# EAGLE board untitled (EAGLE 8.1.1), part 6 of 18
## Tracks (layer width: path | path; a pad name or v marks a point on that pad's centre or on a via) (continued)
S$5547 (continued)
  Bottom 0: 104.1,93.68 104.19,93.45
S$5548
  Bottom 0: 104.19,93.45 56.98,93.45
S$5549
  Bottom 0: 93.36,96.09 95.24,96.09
S$5550
  Bottom 0: 95.24,96.09 95.32,96.1
S$5551
  Bottom 0: 95.32,96.1 95.39,96.14
S$5552
  Bottom 0: 95.39,96.14 95.44,96.19
S$5553
  Bottom 0: 95.44,96.19 95.48,96.27
S$5554
  Bottom 0: 95.48,96.27 95.49,96.34
S$5555
  Bottom 0: 95.49,96.34 95.49,98.22
S$5556
  Bottom 0: 95.49,98.22 95.48,98.3
S$5557
  Bottom 0: 95.48,98.3 95.44,98.37
S$5558
  Bottom 0: 95.44,98.37 95.39,98.42
S$5559
  Bottom 0: 95.39,98.42 95.32,98.47
S$5560
  Bottom 0: 95.32,98.47 95.24,98.48
S$5561
  Bottom 0: 95.24,98.48 93.36,98.48
S$5562
  Bottom 0: 93.36,98.48 93.28,98.47
S$5563
  Bottom 0: 93.28,98.47 93.21,98.42
S$5564
  Bottom 0: 93.21,98.42 93.16,98.37
S$5565
  Bottom 0: 93.16,98.37 93.12,98.3
S$5566
  Bottom 0: 93.12,98.3 93.1,98.22
S$5567
  Bottom 0: 93.1,98.22 93.1,96.34
S$5568
  Bottom 0: 93.1,96.34 93.12,96.27
S$5569
  Bottom 0: 93.12,96.27 93.16,96.19
S$5570
  Bottom 0: 93.16,96.19 93.21,96.14
S$5571
  Bottom 0: 93.21,96.14 93.28,96.1
S$5572
  Bottom 0: 93.28,96.1 93.36,96.09
S$5573
  Bottom 0: 98.59,96.1 98.91,96.12
S$5574
  Bottom 0: 98.91,96.12 99.22,96.22
S$5575
  Bottom 0: 99.22,96.22 99.48,96.41
S$5576
  Bottom 0: 99.48,96.41 99.69,96.67
S$5577
  Bottom 0: 99.69,96.67 99.82,96.97
S$5578
  Bottom 0: 99.82,96.97 99.86,97.29
S$5579
  Bottom 0: 99.86,97.29 99.82,97.61
S$5580
  Bottom 0: 99.82,97.61 99.69,97.91
S$5581
  Bottom 0: 99.69,97.91 99.48,98.16
S$5582
  Bottom 0: 99.48,98.16 99.22,98.35
S$5583
  Bottom 0: 99.22,98.35 98.91,98.45
S$5584
  Bottom 0: 98.91,98.45 98.59,98.48
S$5585
  Bottom 0: 98.59,98.48 98.27,98.41
S$5586
  Bottom 0: 98.27,98.41 97.98,98.26
S$5587
  Bottom 0: 97.98,98.26 97.74,98.04
S$5588
  Bottom 0: 97.74,98.04 97.57,97.77
S$5589
  Bottom 0: 97.57,97.77 97.48,97.45
S$5590
  Bottom 0: 97.48,97.45 97.48,97.12
S$5591
  Bottom 0: 97.48,97.12 97.57,96.81
S$5592
  Bottom 0: 97.57,96.81 97.74,96.53
S$5593
  Bottom 0: 97.74,96.53 97.98,96.31
S$5594
  Bottom 0: 97.98,96.31 98.27,96.16
S$5595
  Bottom 0: 98.27,96.16 98.59,96.1
S$5596
  Bottom 0: 104.8,109.99 105.15,110.05
S$5597
  Bottom 0: 105.15,110.05 105.46,110.2
S$5598
  Bottom 0: 105.46,110.2 105.73,110.42
S$5599
  Bottom 0: 105.73,110.42 105.94,110.71
S$5600
  Bottom 0: 105.94,110.71 106.06,111.03
S$5601
  Bottom 0: 106.06,111.03 106.11,111.38
S$5602
  Bottom 0: 106.11,111.38 106.06,111.72
S$5603
  Bottom 0: 106.06,111.72 105.94,112.05
S$5604
  Bottom 0: 105.94,112.05 105.73,112.33
S$5605
  Bottom 0: 105.73,112.33 105.46,112.56
S$5606
  Bottom 0: 105.46,112.56 105.15,112.71
S$5607
  Bottom 0: 105.15,112.71 104.8,112.77
S$5608
  Bottom 0: 104.8,112.77 104.45,112.75
S$5609
  Bottom 0: 104.45,112.75 104.12,112.64
S$5610
  Bottom 0: 104.12,112.64 104.09,112.63
S$5611
  Bottom 0: 104.09,112.63 103.53,113.2
S$5612
  Bottom 0: 103.53,113.2 103.47,113.24
S$5613
  Bottom 0: 103.47,113.24 103.41,113.28
S$5614
  Bottom 0: 103.41,113.28 103.35,113.3
S$5615
  Bottom 0: 103.35,113.3 103.28,113.32
S$5616
  Bottom 0: 103.28,113.32 103.21,113.33
S$5617
  Bottom 0: 103.21,113.33 98.64,113.33
S$5618
  Bottom 0: 98.64,113.33 98.57,113.46
S$5619
  Bottom 0: 98.57,113.46 98.37,113.67
S$5620
  Bottom 0: 98.37,113.67 98.11,113.83
S$5621
  Bottom 0: 98.11,113.83 97.81,113.89
S$5622
  Bottom 0: 97.81,113.89 97.51,113.87
S$5623
  Bottom 0: 97.51,113.87 97.23,113.76
S$5624
  Bottom 0: 97.23,113.76 96.99,113.57
S$5625
  Bottom 0: 96.99,113.57 96.82,113.33
S$5626
  Bottom 0: 96.82,113.33 96.73,113.03
S$5627
  Bottom 0: 96.73,113.03 96.73,112.73
S$5628
  Bottom 0: 96.73,112.73 96.82,112.44
S$5629
  Bottom 0: 96.82,112.44 96.99,112.19
S$5630
  Bottom 0: 96.99,112.19 97.23,112
S$5631
  Bottom 0: 97.23,112 97.51,111.89
S$5632
  Bottom 0: 97.51,111.89 97.81,111.87
S$5633
  Bottom 0: 97.81,111.87 98.11,111.94
S$5634
  Bottom 0: 98.11,111.94 98.37,112.09
S$5635
  Bottom 0: 98.37,112.09 98.57,112.31
S$5636
  Bottom 0: 98.57,112.31 98.64,112.44
S$5637
  Bottom 0: 98.64,112.44 103.02,112.44
S$5638
  Bottom 0: 103.02,112.44 103.47,111.99
S$5639
  Bottom 0: 103.47,111.99 103.41,111.89
S$5640
  Bottom 0: 103.41,111.89 103.33,111.55
S$5641
  Bottom 0: 103.33,111.55 103.33,111.21
S$5642
  Bottom 0: 103.33,111.21 103.41,110.87
S$5643
  Bottom 0: 103.41,110.87 103.59,110.56
S$5644
  Bottom 0: 103.59,110.56 103.83,110.3
S$5645
  Bottom 0: 103.83,110.3 104.12,110.11
S$5646
  Bottom 0: 104.12,110.11 104.45,110.01
S$5647
  Bottom 0: 104.45,110.01 104.8,109.99
S$5648
  Bottom 0: 85.75,109.99 86.09,110.05
S$5649
  Bottom 0: 86.09,110.05 86.4,110.2
S$5650
  Bottom 0: 86.4,110.2 86.67,110.42
S$5651
  Bottom 0: 86.67,110.42 86.88,110.71
S$5652
  Bottom 0: 86.88,110.71 87.01,111.03
S$5653
  Bottom 0: 87.01,111.03 87.06,111.38
S$5654
  Bottom 0: 87.06,111.38 87.01,111.72
S$5655
  Bottom 0: 87.01,111.72 86.88,112.05
S$5656
  Bottom 0: 86.88,112.05 86.67,112.33
S$5657
  Bottom 0: 86.67,112.33 86.4,112.56
S$5658
  Bottom 0: 86.4,112.56 86.09,112.71
S$5659
  Bottom 0: 86.09,112.71 85.75,112.77
S$5660
  Bottom 0: 85.75,112.77 85.39,112.75
S$5661
  Bottom 0: 85.39,112.75 85.06,112.64
S$5662
  Bottom 0: 85.06,112.64 85.04,112.63
S$5663
  Bottom 0: 85.04,112.63 84.47,113.2
S$5664
  Bottom 0: 84.47,113.2 84.41,113.24
S$5665
  Bottom 0: 84.41,113.24 84.35,113.28
S$5666
  Bottom 0: 84.35,113.28 84.29,113.3
S$5667
  Bottom 0: 84.29,113.3 84.23,113.32
S$5668
  Bottom 0: 84.23,113.32 84.16,113.33
S$5669
  Bottom 0: 84.16,113.33 79.58,113.33
S$5670
  Bottom 0: 79.58,113.33 79.52,113.46
S$5671
  Bottom 0: 79.52,113.46 79.31,113.67
S$5672
  Bottom 0: 79.31,113.67 79.05,113.83
S$5673
  Bottom 0: 79.05,113.83 78.75,113.89
S$5674
  Bottom 0: 78.75,113.89 78.45,113.87
S$5675
  Bottom 0: 78.45,113.87 78.17,113.76
S$5676
  Bottom 0: 78.17,113.76 77.93,113.57
S$5677
  Bottom 0: 77.93,113.57 77.76,113.33
S$5678
  Bottom 0: 77.76,113.33 77.67,113.03
S$5679
  Bottom 0: 77.67,113.03 77.67,112.73
S$5680
  Bottom 0: 77.67,112.73 77.76,112.44
S$5681
  Bottom 0: 77.76,112.44 77.93,112.19
S$5682
  Bottom 0: 77.93,112.19 78.17,112
S$5683
  Bottom 0: 78.17,112 78.45,111.89
S$5684
  Bottom 0: 78.45,111.89 78.75,111.87
S$5685
  Bottom 0: 78.75,111.87 79.05,111.94
S$5686
  Bottom 0: 79.05,111.94 79.31,112.09
S$5687
  Bottom 0: 79.31,112.09 79.52,112.31
S$5688
  Bottom 0: 79.52,112.31 79.58,112.44
S$5689
  Bottom 0: 79.58,112.44 83.97,112.44
S$5690
  Bottom 0: 83.97,112.44 84.41,111.99
S$5691
  Bottom 0: 84.41,111.99 84.36,111.89
S$5692
  Bottom 0: 84.36,111.89 84.27,111.55
S$5693
  Bottom 0: 84.27,111.55 84.27,111.21
S$5694
  Bottom 0: 84.27,111.21 84.36,110.87
S$5695
  Bottom 0: 84.36,110.87 84.53,110.56
S$5696
  Bottom 0: 84.53,110.56 84.77,110.3
S$5697
  Bottom 0: 84.77,110.3 85.06,110.11
S$5698
  Bottom 0: 85.06,110.11 85.39,110.01
S$5699
  Bottom 0: 85.39,110.01 85.75,109.99
S$5700
  Bottom 0: 73.05,112.53 73.39,112.59
S$5701
  Bottom 0: 73.39,112.59 73.7,112.74
S$5702
  Bottom 0: 73.7,112.74 73.97,112.96
S$5703
  Bottom 0: 73.97,112.96 74.18,113.25
S$5704
  Bottom 0: 74.18,113.25 74.31,113.57
S$5705
  Bottom 0: 74.31,113.57 74.36,113.92
S$5706
  Bottom 0: 74.36,113.92 74.31,114.26
S$5707
  Bottom 0: 74.31,114.26 74.18,114.59
S$5708
  Bottom 0: 74.18,114.59 73.97,114.87
S$5709
  Bottom 0: 73.97,114.87 73.7,115.1
S$5710
  Bottom 0: 73.7,115.1 73.39,115.25
S$5711
  Bottom 0: 73.39,115.25 73.05,115.31
S$5712
  Bottom 0: 73.05,115.31 72.69,115.29
S$5713
  Bottom 0: 72.69,115.29 72.36,115.18
S$5714
  Bottom 0: 72.36,115.18 72.07,115
S$5715
  Bottom 0: 72.07,115 71.83,114.74
S$5716
  Bottom 0: 71.83,114.74 71.66,114.43
S$5717
  Bottom 0: 71.66,114.43 71.57,114.09
S$5718
  Bottom 0: 71.57,114.09 71.57,113.75
S$5719
  Bottom 0: 71.57,113.75 71.66,113.41
S$5720
  Bottom 0: 71.66,113.41 71.83,113.1
S$5721
  Bottom 0: 71.83,113.1 72.07,112.84
S$5722
  Bottom 0: 72.07,112.84 72.36,112.65
S$5723
  Bottom 0: 72.36,112.65 72.69,112.55
S$5724
  Bottom 0: 72.69,112.55 73.05,112.53
S$5725
  Bottom 0: 92.09,112.53 92.44,112.59
S$5726
  Bottom 0: 92.44,112.59 92.75,112.74
S$5727
  Bottom 0: 92.75,112.74 93.03,112.96
S$5728
  Bottom 0: 93.03,112.96 93.23,113.25
S$5729
  Bottom 0: 93.23,113.25 93.36,113.57
S$5730
  Bottom 0: 93.36,113.57 93.41,113.92
S$5731
  Bottom 0: 93.41,113.92 93.36,114.26
S$5732
  Bottom 0: 93.36,114.26 93.23,114.59
S$5733
  Bottom 0: 93.23,114.59 93.03,114.87
S$5734
  Bottom 0: 93.03,114.87 92.75,115.1
S$5735
  Bottom 0: 92.75,115.1 92.44,115.25
S$5736
  Bottom 0: 92.44,115.25 92.09,115.31
S$5737
  Bottom 0: 92.09,115.31 91.75,115.29
S$5738
  Bottom 0: 91.75,115.29 91.42,115.18
S$5739
  Bottom 0: 91.42,115.18 91.12,115
S$5740
  Bottom 0: 91.12,115 90.88,114.74
S$5741
  Bottom 0: 90.88,114.74 90.71,114.43
S$5742
  Bottom 0: 90.71,114.43 90.62,114.09
S$5743
  Bottom 0: 90.62,114.09 90.62,113.75
S$5744
  Bottom 0: 90.62,113.75 90.71,113.41
S$5745
  Bottom 0: 90.71,113.41 90.88,113.1
S$5746
  Bottom 0: 90.88,113.1 91.12,112.84
S$5747
  Bottom 0: 91.12,112.84 91.42,112.65
S$5748
  Bottom 0: 91.42,112.65 91.75,112.55
S$5749
  Bottom 0: 91.75,112.55 92.09,112.53
S$5750
  Bottom 0: 88.2,114.17 88.65,114.22
S$5751
  Bottom 0: 88.65,114.22 89.07,114.35
S$5752
  Bottom 0: 89.07,114.35 89.47,114.56
S$5753
  Bottom 0: 89.47,114.56 89.81,114.84
S$5754
  Bottom 0: 89.81,114.84 90.1,115.19
S$5755
  Bottom 0: 90.1,115.19 90.31,115.58
S$5756
  Bottom 0: 90.31,115.58 90.44,116.01
S$5757
  Bottom 0: 90.44,116.01 90.48,116.46
S$5758
  Bottom 0: 90.48,116.46 90.44,116.91
S$5759
  Bottom 0: 90.44,116.91 90.31,117.33
S$5760
  Bottom 0: 90.31,117.33 90.1,117.73
S$5761
  Bottom 0: 90.1,117.73 89.81,118.07
S$5762
  Bottom 0: 89.81,118.07 89.47,118.36
S$5763
  Bottom 0: 89.47,118.36 89.07,118.57
S$5764
  Bottom 0: 89.07,118.57 88.65,118.7
S$5765
  Bottom 0: 88.65,118.7 88.2,118.75
S$5766
  Bottom 0: 88.2,118.75 87.75,118.7
S$5767
  Bottom 0: 87.75,118.7 87.32,118.57
S$5768
  Bottom 0: 87.32,118.57 86.93,118.36
S$5769
  Bottom 0: 86.93,118.36 86.58,118.07
S$5770
  Bottom 0: 86.58,118.07 86.3,117.73
S$5771
  Bottom 0: 86.3,117.73 86.08,117.33
S$5772
  Bottom 0: 86.08,117.33 85.96,116.91
S$5773
  Bottom 0: 85.96,116.91 85.91,116.46
S$5774
  Bottom 0: 85.91,116.46 85.96,116.01
S$5775
  Bottom 0: 85.96,116.01 86.08,115.58
S$5776
  Bottom 0: 86.08,115.58 86.3,115.19
S$5777
  Bottom 0: 86.3,115.19 86.58,114.84
S$5778
  Bottom 0: 86.58,114.84 86.93,114.56
S$5779
  Bottom 0: 86.93,114.56 87.32,114.35
S$5780
  Bottom 0: 87.32,114.35 87.75,114.22
S$5781
  Bottom 0: 87.75,114.22 88.2,114.17
S$5782
  Bottom 0: 88.28,138.54 88.58,138.61
S$5783
  Bottom 0: 88.58,138.61 88.84,138.76
S$5784
  Bottom 0: 88.84,138.76 89.05,138.98
S$5785
  Bottom 0: 89.05,138.98 89.18,139.25
S$5786
  Bottom 0: 89.18,139.25 89.22,139.55
S$5787
  Bottom 0: 89.22,139.55 89.18,139.85
S$5788
  Bottom 0: 89.18,139.85 89.05,140.13
S$5789
  Bottom 0: 89.05,140.13 88.84,140.34
S$5790
  Bottom 0: 88.84,140.34 88.58,140.5
S$5791
  Bottom 0: 88.58,140.5 88.28,140.56
S$5792
  Bottom 0: 88.28,140.56 87.98,140.54
S$5793
  Bottom 0: 87.98,140.54 87.7,140.43
S$5794
  Bottom 0: 87.7,140.43 87.46,140.24
S$5795
  Bottom 0: 87.46,140.24 87.29,140
S$5796
  Bottom 0: 87.29,140 87.2,139.71
S$5797
  Bottom 0: 87.2,139.71 87.2,139.4
S$5798
  Bottom 0: 87.2,139.4 87.29,139.11
S$5799
  Bottom 0: 87.29,139.11 87.46,138.86
S$5800
  Bottom 0: 87.46,138.86 87.7,138.67
S$5801
  Bottom 0: 87.7,138.67 87.98,138.56
S$5802
  Bottom 0: 87.98,138.56 88.28,138.54
S$5803
  Bottom 0: 90.51,148.09 90.86,148.15
S$5804
  Bottom 0: 90.86,148.15 91.17,148.3
S$5805
  Bottom 0: 91.17,148.3 91.44,148.52
S$5806
  Bottom 0: 91.44,148.52 91.65,148.81
S$5807
  Bottom 0: 91.65,148.81 91.78,149.13
S$5808
  Bottom 0: 91.78,149.13 91.82,149.48
S$5809
  Bottom 0: 91.82,149.48 91.78,149.82
S$5810
  Bottom 0: 91.78,149.82 91.65,150.15
S$5811
  Bottom 0: 91.65,150.15 91.44,150.43
S$5812
  Bottom 0: 91.44,150.43 91.17,150.66
S$5813
  Bottom 0: 91.17,150.66 90.86,150.81
S$5814
  Bottom 0: 90.86,150.81 90.51,150.87
S$5815
  Bottom 0: 90.51,150.87 90.16,150.85
S$5816
  Bottom 0: 90.16,150.85 89.83,150.74
S$5817
  Bottom 0: 89.83,150.74 89.53,150.56
S$5818
  Bottom 0: 89.53,150.56 89.29,150.3
S$5819
  Bottom 0: 89.29,150.3 89.12,149.99
S$5820
  Bottom 0: 89.12,149.99 89.04,149.65
S$5821
  Bottom 0: 89.04,149.65 89.04,149.3
S$5822
  Bottom 0: 89.04,149.3 89.12,148.97
S$5823
  Bottom 0: 89.12,148.97 89.29,148.66
S$5824
  Bottom 0: 89.29,148.66 89.53,148.4
S$5825
  Bottom 0: 89.53,148.4 89.83,148.21
S$5826
  Bottom 0: 89.83,148.21 90.16,148.11
S$5827
  Bottom 0: 90.16,148.11 90.51,148.09
S$5828
  Bottom 0: 246.64,93.68 239.2,101.12
S$5829
  Bottom 0: 239.2,101.12 239.21,101.15
S$5830
  Bottom 0: 239.21,101.15 239.26,101.45
S$5831
  Bottom 0: 239.26,101.45 239.21,101.75
S$5832
  Bottom 0: 239.21,101.75 239.08,102.02
S$5833
  Bottom 0: 239.08,102.02 238.88,102.24
S$5834
  Bottom 0: 238.88,102.24 238.61,102.39
S$5835
  Bottom 0: 238.61,102.39 238.32,102.46
S$5836
  Bottom 0: 238.32,102.46 238.08,102.44
S$5837
  Bottom 0: 238.08,102.44 246.78,111.14
S$5838
  Bottom 0: 246.78,111.14 246.82,111.19
S$5839
  Bottom 0: 246.82,111.19 246.86,111.25
S$5840
  Bottom 0: 246.86,111.25 246.88,111.31
S$5841
  Bottom 0: 246.88,111.31 246.9,111.38
S$5842
  Bottom 0: 246.9,111.38 246.9,111.45
S$5843
  Bottom 0: 246.9,111.45 246.9,138.72
S$5844
  Bottom 0: 246.9,138.72 246.97,138.78
S$5845
  Bottom 0: 246.97,138.78 247.1,138.99
S$5846
  Bottom 0: 247.1,138.99 247.15,139.24
S$5847
  Bottom 0: 247.15,139.24 247.1,139.49
S$5848
  Bottom 0: 247.1,139.49 246.97,139.7
S$5849
  Bottom 0: 246.97,139.7 246.77,139.85
S$5850
  Bottom 0: 246.77,139.85 246.52,139.92
S$5851
  Bottom 0: 246.52,139.92 246.27,139.9
S$5852
  Bottom 0: 246.27,139.9 246.05,139.78
S$5853
  Bottom 0: 246.05,139.78 245.88,139.6
S$5854
  Bottom 0: 245.88,139.6 245.79,139.37
S$5855
  Bottom 0: 245.79,139.37 245.79,139.11
S$5856
  Bottom 0: 245.79,139.11 245.88,138.88
S$5857
  Bottom 0: 245.88,138.88 246.02,138.72
S$5858
  Bottom 0: 246.02,138.72 246.02,111.64
S$5859
  Bottom 0: 246.02,111.64 229.12,94.74
S$5860
  Bottom 0: 229.12,94.74 229.14,94.87
S$5861
  Bottom 0: 229.14,94.87 229.09,95.21
S$5862
  Bottom 0: 229.09,95.21 228.97,95.54
S$5863
  Bottom 0: 228.97,95.54 228.75,95.82
S$5864
  Bottom 0: 228.75,95.82 228.49,96.05
S$5865
  Bottom 0: 228.49,96.05 228.18,96.19
S$5866
  Bottom 0: 228.18,96.19 228.18,97.27
S$5867
  Bottom 0: 228.18,97.27 228.18,97.34
S$5868
  Bottom 0: 228.18,97.34 228.16,97.41
S$5869
  Bottom 0: 228.16,97.41 228.14,97.47
S$5870
  Bottom 0: 228.14,97.47 228.1,97.53
S$5871
  Bottom 0: 228.1,97.53 228.05,97.59
S$5872
  Bottom 0: 228.05,97.59 225.4,100.25
S$5873
  Bottom 0: 225.4,100.25 243.96,118.81
S$5874
  Bottom 0: 243.96,118.81 244,118.87
S$5875
  Bottom 0: 244,118.87 244.04,118.93
S$5876
  Bottom 0: 244.04,118.93 244.06,118.99
S$5877
  Bottom 0: 244.06,118.99 244.08,119.06
S$5878
  Bottom 0: 244.08,119.06 244.08,119.13
S$5879
  Bottom 0: 244.08,119.13 244.08,140.04
S$5880
  Bottom 0: 244.08,140.04 244.08,140.12
S$5881
  Bottom 0: 244.08,140.12 244.06,140.18
S$5882
  Bottom 0: 244.06,140.18 244.04,140.24
S$5883
  Bottom 0: 244.04,140.24 244,140.31
S$5884
  Bottom 0: 244,140.31 243.96,140.36
S$5885
  Bottom 0: 243.96,140.36 231.98,152.33
S$5886
  Bottom 0: 231.98,152.33 231.93,152.38
S$5887
  Bottom 0: 231.93,152.38 231.86,152.41
S$5888
  Bottom 0: 231.86,152.41 231.8,152.44
S$5889
  Bottom 0: 231.8,152.44 231.74,152.46
S$5890
  Bottom 0: 231.74,152.46 231.67,152.46
S$5891
  Bottom 0: 231.67,152.46 231.44,152.46
S$5892
  Bottom 0: 231.44,152.46 231.35,152.69
S$5893
  Bottom 0: 231.35,152.69 231.14,152.97
S$5894
  Bottom 0: 231.14,152.97 230.87,153.2
S$5895
  Bottom 0: 230.87,153.2 230.56,153.35
S$5896
  Bottom 0: 230.56,153.35 230.21,153.41
S$5897
  Bottom 0: 230.21,153.41 229.86,153.39
S$5898
  Bottom 0: 229.86,153.39 229.53,153.28
S$5899
  Bottom 0: 229.53,153.28 229.24,153.1
S$5900
  Bottom 0: 229.24,153.1 229,152.84
S$5901
  Bottom 0: 229,152.84 228.82,152.53
S$5902
  Bottom 0: 228.82,152.53 228.8,152.46
S$5903
  Bottom 0: 228.8,152.46 227.22,152.46
S$5904
  Bottom 0: 227.22,152.46 227.58,152.66
S$5905
  Bottom 0: 227.58,152.66 227.93,152.94
S$5906
  Bottom 0: 227.93,152.94 228.21,153.29
S$5907
  Bottom 0: 228.21,153.29 228.43,153.68
S$5908
  Bottom 0: 228.43,153.68 228.55,154.11
S$5909
  Bottom 0: 228.55,154.11 228.6,154.56
S$5910
  Bottom 0: 228.6,154.56 228.55,155.01
S$5911
  Bottom 0: 228.55,155.01 228.43,155.43
S$5912
  Bottom 0: 228.43,155.43 228.21,155.83
S$5913
  Bottom 0: 228.21,155.83 227.93,156.17
S$5914
  Bottom 0: 227.93,156.17 227.58,156.46
S$5915
  Bottom 0: 227.58,156.46 227.19,156.67
S$5916
  Bottom 0: 227.19,156.67 226.76,156.8
S$5917
  Bottom 0: 226.76,156.8 226.31,156.84
S$5918
  Bottom 0: 226.31,156.84 225.87,156.8
S$5919
  Bottom 0: 225.87,156.8 225.44,156.67
S$5920
  Bottom 0: 225.44,156.67 225.04,156.46
S$5921
  Bottom 0: 225.04,156.46 224.7,156.17
S$5922
  Bottom 0: 224.7,156.17 224.41,155.83
S$5923
  Bottom 0: 224.41,155.83 224.2,155.43
S$5924
  Bottom 0: 224.2,155.43 224.07,155.01
S$5925
  Bottom 0: 224.07,155.01 224.03,154.56
S$5926
  Bottom 0: 224.03,154.56 224.07,154.11
S$5927
  Bottom 0: 224.07,154.11 224.2,153.68
S$5928
  Bottom 0: 224.2,153.68 224.41,153.29
S$5929
  Bottom 0: 224.41,153.29 224.7,152.94
S$5930
  Bottom 0: 224.7,152.94 225.04,152.66
S$5931
  Bottom 0: 225.04,152.66 225.41,152.46
S$5932
  Bottom 0: 225.41,152.46 217.72,152.46
S$5933
  Bottom 0: 217.72,152.46 211.52,158.66
S$5934
  Bottom 0: 211.52,158.66 211.47,158.7
S$5935
  Bottom 0: 211.47,158.7 211.4,158.74
S$5936
  Bottom 0: 211.4,158.74 211.34,158.76
S$5937
  Bottom 0: 211.34,158.76 211.28,158.78
S$5938
  Bottom 0: 211.28,158.78 211.21,158.79
S$5939
  Bottom 0: 211.21,158.79 209.29,158.79
S$5940
  Bottom 0: 209.29,158.79 209.49,159.02
S$5941
  Bottom 0: 209.49,159.02 209.63,159.32
S$5942
  Bottom 0: 209.63,159.32 209.68,159.64
S$5943
  Bottom 0: 209.68,159.64 209.63,159.96
S$5944
  Bottom 0: 209.63,159.96 209.49,160.26
S$5945
  Bottom 0: 209.49,160.26 209.28,160.5
S$5946
  Bottom 0: 209.28,160.5 209.1,160.62
S$5947
  Bottom 0: 209.1,160.62 209.1,161.66
S$5948
  Bottom 0: 209.1,161.66 209.1,161.75
S$5949
  Bottom 0: 209.1,161.75 209.08,161.84
S$5950
  Bottom 0: 209.08,161.84 209.04,161.92
S$5951
  Bottom 0: 209.04,161.92 209,162
S$5952
  Bottom 0: 209,162 208.94,162.06
S$5953
  Bottom 0: 208.94,162.06 201.29,169.7
S$5954
  Bottom 0: 201.29,169.7 201.63,169.68
S$5955
  Bottom 0: 201.63,169.68 201.98,169.74
S$5956
  Bottom 0: 201.98,169.74 202.16,169.83
S$5957
  Bottom 0: 202.16,169.83 205.24,166.75
S$5958
  Bottom 0: 205.24,166.75 205.29,166.71
S$5959
  Bottom 0: 205.29,166.71 205.35,166.66
S$5960
  Bottom 0: 205.35,166.66 205.41,166.64
S$5961
  Bottom 0: 205.41,166.64 205.48,166.62
S$5962
  Bottom 0: 205.48,166.62 205.55,166.62
S$5963
  Bottom 0: 205.55,166.62 208.77,166.62
S$5964
  Bottom 0: 208.77,166.62 211.33,164.06
S$5965
  Bottom 0: 211.33,164.06 211.01,164.08
S$5966
  Bottom 0: 211.01,164.08 210.69,164.02
S$5967
  Bottom 0: 210.69,164.02 210.4,163.87
S$5968
  Bottom 0: 210.4,163.87 210.17,163.65
S$5969
  Bottom 0: 210.17,163.65 210,163.37
S$5970
  Bottom 0: 210,163.37 209.91,163.06
S$5971
  Bottom 0: 209.91,163.06 209.91,162.73
S$5972
  Bottom 0: 209.91,162.73 210,162.42
S$5973
  Bottom 0: 210,162.42 210.17,162.14
S$5974
  Bottom 0: 210.17,162.14 210.4,161.92
S$5975
  Bottom 0: 210.4,161.92 210.69,161.77
S$5976
  Bottom 0: 210.69,161.77 211.01,161.71
S$5977
  Bottom 0: 211.01,161.71 211.34,161.73
S$5978
  Bottom 0: 211.34,161.73 211.64,161.83
S$5979
  Bottom 0: 211.64,161.83 211.91,162.02
S$5980
  Bottom 0: 211.91,162.02 212.11,162.28
S$5981
  Bottom 0: 212.11,162.28 212.24,162.57
S$5982
  Bottom 0: 212.24,162.57 212.29,162.89
S$5983
  Bottom 0: 212.29,162.89 212.24,163.22
S$5984
  Bottom 0: 212.24,163.22 212.23,163.25
S$5985
  Bottom 0: 212.23,163.25 212.28,163.24
S$5986
  Bottom 0: 212.28,163.24 212.35,163.23
S$5987
  Bottom 0: 212.35,163.23 213.16,163.23
S$5988
  Bottom 0: 213.16,163.23 216.78,159.61
S$5989
  Bottom 0: 216.78,159.61 216.58,159.59
S$5990
  Bottom 0: 216.58,159.59 216.3,159.48
S$5991
  Bottom 0: 216.3,159.48 216.06,159.29
S$5992
  Bottom 0: 216.06,159.29 215.89,159.04
S$5993
  Bottom 0: 215.89,159.04 215.8,158.75
S$5994
  Bottom 0: 215.8,158.75 215.8,158.45
S$5995
  Bottom 0: 215.8,158.45 215.89,158.16
S$5996
  Bottom 0: 215.89,158.16 216.06,157.91
S$5997
  Bottom 0: 216.06,157.91 216.3,157.72
S$5998
  Bottom 0: 216.3,157.72 216.58,157.61
S$5999
  Bottom 0: 216.58,157.61 216.88,157.59
S$6000
  Bottom 0: 216.88,157.59 217.18,157.66
S$6001
  Bottom 0: 217.18,157.66 217.44,157.81
S$6002
  Bottom 0: 217.44,157.81 217.64,158.03
S$6003
  Bottom 0: 217.64,158.03 217.78,158.3
S$6004
  Bottom 0: 217.78,158.3 217.81,158.57
S$6005
  Bottom 0: 217.81,158.57 218.98,157.4
S$6006
  Bottom 0: 218.98,157.4 219.03,157.36
S$6007
  Bottom 0: 219.03,157.36 219.09,157.32
S$6008
  Bottom 0: 219.09,157.32 219.16,157.29
S$6009
  Bottom 0: 219.16,157.29 219.22,157.28
S$6010
  Bottom 0: 219.22,157.28 219.29,157.27
S$6011
  Bottom 0: 219.29,157.27 235.43,157.27
S$6012
  Bottom 0: 235.43,157.27 241,151.7
S$6013
  Bottom 0: 241,151.7 241.05,151.66
S$6014
  Bottom 0: 241.05,151.66 241.11,151.62
S$6015
  Bottom 0: 241.11,151.62 241.17,151.6
S$6016
  Bottom 0: 241.17,151.6 241.24,151.58
S$6017
  Bottom 0: 241.24,151.58 241.31,151.58
S$6018
  Bottom 0: 241.31,151.58 247.85,151.58
S$6019
  Bottom 0: 247.85,151.58 247.87,151.51
S$6020
  Bottom 0: 247.87,151.51 248.05,151.2
S$6021
  Bottom 0: 248.05,151.2 248.28,150.94
S$6022
  Bottom 0: 248.28,150.94 248.58,150.75
S$6023
  Bottom 0: 248.58,150.75 248.91,150.65
S$6024
  Bottom 0: 248.91,150.65 249.26,150.63
S$6025
  Bottom 0: 249.26,150.63 249.61,150.69
S$6026
  Bottom 0: 249.61,150.69 249.79,150.77
S$6027
  Bottom 0: 249.79,150.77 249.88,150.68
S$6028
  Bottom 0: 249.88,150.68 249.94,150.63
S$6029
  Bottom 0: 249.94,150.63 250,150.6
S$6030
  Bottom 0: 250,150.6 250.06,150.57
S$6031
  Bottom 0: 250.06,150.57 250.13,150.56
S$6032
  Bottom 0: 250.13,150.56 250.2,150.55
S$6033
  Bottom 0: 250.2,150.55 252.78,150.55
S$6034
  Bottom 0: 252.78,150.55 253.72,149.61
S$6035
  Bottom 0: 253.72,149.61 253.5,149.6
S$6036
  Bottom 0: 253.5,149.6 253.22,149.48
S$6037
  Bottom 0: 253.22,149.48 252.98,149.3
S$6038
  Bottom 0: 252.98,149.3 252.81,149.04
S$6039
  Bottom 0: 252.81,149.04 244.14,149.04
S$6040
  Bottom 0: 244.14,149.04 244.18,149.13
S$6041
  Bottom 0: 244.18,149.13 244.22,149.48
S$6042
  Bottom 0: 244.22,149.48 244.18,149.82
S$6043
  Bottom 0: 244.18,149.82 244.05,150.15
S$6044
  Bottom 0: 244.05,150.15 243.84,150.43
S$6045
  Bottom 0: 243.84,150.43 243.57,150.66
S$6046
  Bottom 0: 243.57,150.66 243.26,150.81
S$6047
  Bottom 0: 243.26,150.81 242.91,150.87
S$6048
  Bottom 0: 242.91,150.87 242.56,150.85
S$6049
  Bottom 0: 242.56,150.85 242.23,150.74
S$6050
  Bottom 0: 242.23,150.74 241.94,150.56
S$6051
  Bottom 0: 241.94,150.56 241.7,150.3
S$6052
  Bottom 0: 241.7,150.3 241.52,149.99
S$6053
  Bottom 0: 241.52,149.99 241.44,149.65
S$6054
  Bottom 0: 241.44,149.65 241.44,149.3
S$6055
  Bottom 0: 241.44,149.3 241.52,148.97
S$6056
  Bottom 0: 241.52,148.97 241.7,148.66
S$6057
  Bottom 0: 241.7,148.66 241.94,148.4
S$6058
  Bottom 0: 241.94,148.4 242.23,148.21
S$6059
  Bottom 0: 242.23,148.21 242.56,148.11
S$6060
  Bottom 0: 242.56,148.11 242.91,148.09
S$6061
  Bottom 0: 242.91,148.09 243.26,148.15
S$6062
  Bottom 0: 243.26,148.15 243.45,148.25
S$6063
  Bottom 0: 243.45,148.25 243.5,148.21
S$6064
  Bottom 0: 243.5,148.21 243.56,148.18
S$6065
  Bottom 0: 243.56,148.18 243.63,148.17
S$6066
  Bottom 0: 243.63,148.17 243.7,148.16
S$6067
  Bottom 0: 243.7,148.16 252.81,148.16
S$6068
  Bottom 0: 252.81,148.16 252.98,147.91
S$6069
  Bottom 0: 252.98,147.91 253.22,147.73
S$6070
  Bottom 0: 253.22,147.73 253.5,147.62
S$6071
  Bottom 0: 253.5,147.62 253.8,147.59
S$6072
  Bottom 0: 253.8,147.59 254.1,147.66
S$6073
  Bottom 0: 254.1,147.66 254.36,147.81
S$6074
  Bottom 0: 254.36,147.81 254.56,148.03
S$6075
  Bottom 0: 254.56,148.03 254.7,148.31
S$6076
  Bottom 0: 254.7,148.31 254.74,148.59
S$6077
  Bottom 0: 254.74,148.59 257.62,145.71
S$6078
  Bottom 0: 257.62,145.71 248.02,136.09
S$6079
  Bottom 0: 248.02,136.09 247.97,136.03
S$6080
  Bottom 0: 247.97,136.03 247.93,135.97
S$6081
  Bottom 0: 247.93,135.97 247.91,135.91
S$6082
  Bottom 0: 247.91,135.91 247.89,135.85
S$6083
  Bottom 0: 247.89,135.85 247.89,135.78
S$6084
  Bottom 0: 247.89,135.78 247.89,127
S$6085
  Bottom 0: 247.89,127 247.75,126.84
S$6086
  Bottom 0: 247.75,126.84 247.66,126.61
S$6087
  Bottom 0: 247.66,126.61 247.66,126.36
S$6088
  Bottom 0: 247.66,126.36 247.75,126.12
S$6089
  Bottom 0: 247.75,126.12 247.89,125.97
S$6090
  Bottom 0: 247.89,125.97 247.89,109.06
S$6091
  Bottom 0: 247.89,109.06 244.91,106.09
S$6092
  Bottom 0: 244.91,106.09 244.86,106.03
S$6093
  Bottom 0: 244.86,106.03 244.83,105.97
S$6094
  Bottom 0: 244.83,105.97 244.79,105.91
S$6095
  Bottom 0: 244.79,105.91 244.78,105.84
S$6096
  Bottom 0: 244.78,105.84 244.78,105.77
S$6097
  Bottom 0: 244.78,105.77 244.78,101.33
S$6098
  Bottom 0: 244.78,101.33 244.78,101.25
S$6099
  Bottom 0: 244.78,101.25 244.79,101.19
S$6100
  Bottom 0: 244.79,101.19 244.83,101.12
S$6101
  Bottom 0: 244.83,101.12 244.86,101.07
S$6102
  Bottom 0: 244.86,101.07 244.91,101.01
S$6103
  Bottom 0: 244.91,101.01 245.57,100.34
S$6104
  Bottom 0: 245.57,100.34 245.63,100.3
S$6105
  Bottom 0: 245.63,100.3 245.69,100.26
S$6106
  Bottom 0: 245.69,100.26 245.75,100.24
S$6107
  Bottom 0: 245.75,100.24 245.82,100.22
S$6108
  Bottom 0: 245.82,100.22 245.89,100.22
S$6109
  Bottom 0: 245.89,100.22 247.83,100.22
S$6110
  Bottom 0: 247.83,100.22 248.48,99.56
S$6111
  Bottom 0: 248.48,99.56 248.19,99.65
S$6112
  Bottom 0: 248.19,99.65 247.75,99.69
S$6113
  Bottom 0: 247.75,99.69 247.3,99.65
S$6114
  Bottom 0: 247.3,99.65 246.87,99.52
S$6115
  Bottom 0: 246.87,99.52 246.48,99.31
S$6116
  Bottom 0: 246.48,99.31 246.13,99.02
S$6117
  Bottom 0: 246.13,99.02 245.85,98.68
S$6118
  Bottom 0: 245.85,98.68 245.63,98.28
S$6119
  Bottom 0: 245.63,98.28 245.51,97.86
S$6120
  Bottom 0: 245.51,97.86 245.46,97.41
S$6121
  Bottom 0: 245.46,97.41 245.51,96.96
S$6122
  Bottom 0: 245.51,96.96 245.63,96.53
S$6123
  Bottom 0: 245.63,96.53 245.85,96.14
S$6124
  Bottom 0: 245.85,96.14 246.13,95.79
S$6125
  Bottom 0: 246.13,95.79 246.48,95.51
S$6126
  Bottom 0: 246.48,95.51 246.87,95.3
S$6127
  Bottom 0: 246.87,95.3 247.3,95.17
S$6128
  Bottom 0: 247.3,95.17 247.75,95.12
S$6129
  Bottom 0: 247.75,95.12 248.19,95.17
S$6130
  Bottom 0: 248.19,95.17 248.62,95.3
S$6131
  Bottom 0: 248.62,95.3 249.02,95.51
S$6132
  Bottom 0: 249.02,95.51 249.36,95.79
S$6133
  Bottom 0: 249.36,95.79 249.64,96.14
S$6134
  Bottom 0: 249.64,96.14 249.86,96.53
S$6135
  Bottom 0: 249.86,96.53 249.99,96.96
S$6136
  Bottom 0: 249.99,96.96 250.03,97.41
S$6137
  Bottom 0: 250.03,97.41 249.99,97.86
S$6138
  Bottom 0: 249.99,97.86 249.9,98.15
S$6139
  Bottom 0: 249.9,98.15 251.12,96.93
S$6140
  Bottom 0: 251.12,96.93 251.12,96.19
S$6141
  Bottom 0: 251.12,96.19 250.96,96.13
S$6142
  Bottom 0: 250.96,96.13 250.67,95.95
S$6143
  Bottom 0: 250.67,95.95 250.43,95.69
S$6144
  Bottom 0: 250.43,95.69 250.26,95.38
S$6145
  Bottom 0: 250.26,95.38 250.17,95.04
S$6146
  Bottom 0: 250.17,95.04 250.17,94.7
S$6147
  Bottom 0: 250.17,94.7 250.26,94.36
S$6148
  Bottom 0: 250.26,94.36 250.43,94.05
S$6149
  Bottom 0: 250.43,94.05 250.67,93.79
S$6150
  Bottom 0: 250.67,93.79 250.84,93.68
S$6151
  Bottom 0: 250.84,93.68 246.64,93.68
S$6152
  Bottom 0: 252.28,93.68 252.3,93.69
S$6153
  Bottom 0: 252.3,93.69 252.57,93.91
S$6154
  Bottom 0: 252.57,93.91 252.78,94.2
S$6155
  Bottom 0: 252.78,94.2 252.91,94.52
S$6156
  Bottom 0: 252.91,94.52 252.95,94.87
S$6157
  Bottom 0: 252.95,94.87 252.91,95.21
S$6158
  Bottom 0: 252.91,95.21 252.78,95.54
S$6159
  Bottom 0: 252.78,95.54 252.57,95.82
S$6160
  Bottom 0: 252.57,95.82 252.3,96.05
S$6161
  Bottom 0: 252.3,96.05 252,96.19
S$6162
  Bottom 0: 252,96.19 252,97.12
S$6163
  Bottom 0: 252,97.12 251.99,97.19
S$6164
  Bottom 0: 251.99,97.19 251.98,97.26
S$6165
  Bottom 0: 251.98,97.26 251.95,97.32
S$6166
  Bottom 0: 251.95,97.32 251.91,97.38
S$6167
  Bottom 0: 251.91,97.38 251.87,97.43
S$6168
  Bottom 0: 251.87,97.43 248.53,100.78
S$6169
  Bottom 0: 248.53,100.78 254.93,100.78
S$6170
  Bottom 0: 254.93,100.78 255,100.78
S$6171
  Bottom 0: 255,100.78 255.06,100.8
S$6172
  Bottom 0: 255.06,100.8 255.12,100.82
S$6173
  Bottom 0: 255.12,100.82 255.18,100.86
S$6174
  Bottom 0: 255.18,100.86 255.24,100.9
S$6175
  Bottom 0: 255.24,100.9 255.65,101.31
S$6176
  Bottom 0: 255.65,101.31 255.71,101.28
S$6177
  Bottom 0: 255.71,101.28 256.03,101.21
S$6178
  Bottom 0: 256.03,101.21 256.35,101.23
S$6179
  Bottom 0: 256.35,101.23 256.66,101.34
S$6180
  Bottom 0: 256.66,101.34 256.92,101.53
S$6181
  Bottom 0: 256.92,101.53 257.13,101.78
S$6182
  Bottom 0: 257.13,101.78 257.26,102.08
S$6183
  Bottom 0: 257.26,102.08 257.3,102.4
S$6184
  Bottom 0: 257.3,102.4 257.26,102.72
S$6185
  Bottom 0: 257.26,102.72 257.13,103.02
S$6186
  Bottom 0: 257.13,103.02 256.92,103.28
S$6187
  Bottom 0: 256.92,103.28 256.66,103.46
S$6188
  Bottom 0: 256.66,103.46 256.35,103.57
S$6189
  Bottom 0: 256.35,103.57 256.03,103.59
S$6190
  Bottom 0: 256.03,103.59 255.71,103.53
S$6191
  Bottom 0: 255.71,103.53 255.42,103.38
S$6192
  Bottom 0: 255.42,103.38 255.18,103.15
S$6193
  Bottom 0: 255.18,103.15 255.01,102.88
S$6194
  Bottom 0: 255.01,102.88 254.93,102.56
S$6195
  Bottom 0: 254.93,102.56 254.93,102.24
S$6196
  Bottom 0: 254.93,102.24 255.01,101.94
S$6197
  Bottom 0: 255.01,101.94 254.74,101.66
S$6198
  Bottom 0: 254.74,101.66 249.79,101.66
S$6199
  Bottom 0: 249.79,101.66 249.98,101.87
S$6200
  Bottom 0: 249.98,101.87 250.11,102.17
S$6201
  Bottom 0: 250.11,102.17 250.16,102.49
S$6202
  Bottom 0: 250.16,102.49 250.11,102.81
S$6203
  Bottom 0: 250.11,102.81 249.98,103.11
S$6204
  Bottom 0: 249.98,103.11 249.76,103.35
S$6205
  Bottom 0: 249.76,103.35 249.58,103.47
S$6206
  Bottom 0: 249.58,103.47 249.58,111.78
S$6207
  Bottom 0: 249.58,111.78 255.18,117.38
S$6208
  Bottom 0: 255.18,117.38 255.16,117.33
S$6209
  Bottom 0: 255.16,117.33 255.03,116.91
S$6210
  Bottom 0: 255.03,116.91 254.99,116.46
S$6211
  Bottom 0: 254.99,116.46 255.03,116.01
S$6212
  Bottom 0: 255.03,116.01 255.16,115.58
S$6213
  Bottom 0: 255.16,115.58 255.37,115.19
S$6214
  Bottom 0: 255.37,115.19 255.66,114.84
S$6215
  Bottom 0: 255.66,114.84 256,114.56
S$6216
  Bottom 0: 256,114.56 256.4,114.35
S$6217
  Bottom 0: 256.4,114.35 256.82,114.22
S$6218
  Bottom 0: 256.82,114.22 257.27,114.17
S$6219
  Bottom 0: 257.27,114.17 257.72,114.22
S$6220
  Bottom 0: 257.72,114.22 258.14,114.35
S$6221
  Bottom 0: 258.14,114.35 258.54,114.56
S$6222
  Bottom 0: 258.54,114.56 258.89,114.84
S$6223
  Bottom 0: 258.89,114.84 259.17,115.19
S$6224
  Bottom 0: 259.17,115.19 259.38,115.58
S$6225
  Bottom 0: 259.38,115.58 259.51,116.01
S$6226
  Bottom 0: 259.51,116.01 259.56,116.46
S$6227
  Bottom 0: 259.56,116.46 259.51,116.91
S$6228
  Bottom 0: 259.51,116.91 259.38,117.33
S$6229
  Bottom 0: 259.38,117.33 259.17,117.73
S$6230
  Bottom 0: 259.17,117.73 258.89,118.07
S$6231
  Bottom 0: 258.89,118.07 258.54,118.36
S$6232
  Bottom 0: 258.54,118.36 258.14,118.57
S$6233
  Bottom 0: 258.14,118.57 257.72,118.7
S$6234
  Bottom 0: 257.72,118.7 257.27,118.75
S$6235
  Bottom 0: 257.27,118.75 256.82,118.7
S$6236
  Bottom 0: 256.82,118.7 256.4,118.57
S$6237
  Bottom 0: 256.4,118.57 256.35,118.55
S$6238
  Bottom 0: 256.35,118.55 258.25,120.45
S$6239
  Bottom 0: 258.25,120.45 258.38,120.41
S$6240
  Bottom 0: 258.38,120.41 258.7,120.41
S$6241
  Bottom 0: 258.7,120.41 259.01,120.5
S$6242
  Bottom 0: 259.01,120.5 259.29,120.67
S$6243
  Bottom 0: 259.29,120.67 259.5,120.92
S$6244
  Bottom 0: 259.5,120.92 259.64,121.22
S$6245
  Bottom 0: 259.64,121.22 259.69,121.54
S$6246
  Bottom 0: 259.69,121.54 259.64,121.86
S$6247
  Bottom 0: 259.64,121.86 259.5,122.16
S$6248
  Bottom 0: 259.5,122.16 259.29,122.4
S$6249
  Bottom 0: 259.29,122.4 259.01,122.58
S$6250
  Bottom 0: 259.01,122.58 258.7,122.67
S$6251
  Bottom 0: 258.7,122.67 258.38,122.67
S$6252
  Bottom 0: 258.38,122.67 258.25,122.63
S$6253
  Bottom 0: 258.25,122.63 258.2,122.68
S$6254
  Bottom 0: 258.2,122.68 258.2,129.9
S$6255
  Bottom 0: 258.2,129.9 258.36,129.61
S$6256
  Bottom 0: 258.36,129.61 258.6,129.35
S$6257
  Bottom 0: 258.6,129.35 258.9,129.16
S$6258
  Bottom 0: 258.9,129.16 259.23,129.06
S$6259
  Bottom 0: 259.23,129.06 259.58,129.04
S$6260
  Bottom 0: 259.58,129.04 259.92,129.1
S$6261
  Bottom 0: 259.92,129.1 260.24,129.25
S$6262
  Bottom 0: 260.24,129.25 260.5,129.47
S$6263
  Bottom 0: 260.5,129.47 260.72,129.76
S$6264
  Bottom 0: 260.72,129.76 260.84,130.08
S$6265
  Bottom 0: 260.84,130.08 260.89,130.43
S$6266
  Bottom 0: 260.89,130.43 260.84,130.77
S$6267
  Bottom 0: 260.84,130.77 260.72,131.1
S$6268
  Bottom 0: 260.72,131.1 260.5,131.38
S$6269
  Bottom 0: 260.5,131.38 260.24,131.61
S$6270
  Bottom 0: 260.24,131.61 259.92,131.76
S$6271
  Bottom 0: 259.92,131.76 259.58,131.82
S$6272
  Bottom 0: 259.58,131.82 259.23,131.8
S$6273
  Bottom 0: 259.23,131.8 258.9,131.69
S$6274
  Bottom 0: 258.9,131.69 258.6,131.51
S$6275
  Bottom 0: 258.6,131.51 258.36,131.25
S$6276
  Bottom 0: 258.36,131.25 258.2,130.96
S$6277
  Bottom 0: 258.2,130.96 258.2,134.69
S$6278
  Bottom 0: 258.2,134.69 259.94,136.43
S$6279
  Bottom 0: 259.94,136.43 259.92,136.38
S$6280
  Bottom 0: 259.92,136.38 259.79,135.96
S$6281
  Bottom 0: 259.79,135.96 259.74,135.51
S$6282
  Bottom 0: 259.74,135.51 259.79,135.06
S$6283
  Bottom 0: 259.79,135.06 259.92,134.63
S$6284
  Bottom 0: 259.92,134.63 260.13,134.24
S$6285
  Bottom 0: 260.13,134.24 260.42,133.89
S$6286
  Bottom 0: 260.42,133.89 260.76,133.61
S$6287
  Bottom 0: 260.76,133.61 261.16,133.4
S$6288
  Bottom 0: 261.16,133.4 261.58,133.27
S$6289
  Bottom 0: 261.58,133.27 262.03,133.22
S$6290
  Bottom 0: 262.03,133.22 262.48,133.27
S$6291
  Bottom 0: 262.48,133.27 262.9,133.4
S$6292
  Bottom 0: 262.9,133.4 263.3,133.61
S$6293
  Bottom 0: 263.3,133.61 263.65,133.89
S$6294
  Bottom 0: 263.65,133.89 263.93,134.24
S$6295
  Bottom 0: 263.93,134.24 264.14,134.63
S$6296
  Bottom 0: 264.14,134.63 264.27,135.06
S$6297
  Bottom 0: 264.27,135.06 264.31,135.51
S$6298
  Bottom 0: 264.31,135.51 264.27,135.96
S$6299
  Bottom 0: 264.27,135.96 264.14,136.38
S$6300
  Bottom 0: 264.14,136.38 263.93,136.78
S$6301
  Bottom 0: 263.93,136.78 263.65,137.12
S$6302
  Bottom 0: 263.65,137.12 263.3,137.41
S$6303
  Bottom 0: 263.3,137.41 262.9,137.62
S$6304
  Bottom 0: 262.9,137.62 262.48,137.75
S$6305
  Bottom 0: 262.48,137.75 262.03,137.79
S$6306
  Bottom 0: 262.03,137.79 261.58,137.75
S$6307
  Bottom 0: 261.58,137.75 261.16,137.62
S$6308
  Bottom 0: 261.16,137.62 261.11,137.6
S$6309
  Bottom 0: 261.11,137.6 263.01,139.5
S$6310
  Bottom 0: 263.01,139.5 263.14,139.46
S$6311
  Bottom 0: 263.14,139.46 263.46,139.46
S$6312
  Bottom 0: 263.46,139.46 263.77,139.55
S$6313
  Bottom 0: 263.77,139.55 264.05,139.72
S$6314
  Bottom 0: 264.05,139.72 264.26,139.97
S$6315
  Bottom 0: 264.26,139.97 264.4,140.27
S$6316
  Bottom 0: 264.4,140.27 264.44,140.59
S$6317
  Bottom 0: 264.44,140.59 264.4,140.91
S$6318
  Bottom 0: 264.4,140.91 264.26,141.21
S$6319
  Bottom 0: 264.26,141.21 264.05,141.45
S$6320
  Bottom 0: 264.05,141.45 263.77,141.63
S$6321
  Bottom 0: 263.77,141.63 263.46,141.72
S$6322
  Bottom 0: 263.46,141.72 263.14,141.72
S$6323
  Bottom 0: 263.14,141.72 262.83,141.63
S$6324
  Bottom 0: 262.83,141.63 262.56,141.45
S$6325
  Bottom 0: 262.56,141.45 262.34,141.21
S$6326
  Bottom 0: 262.34,141.21 262.2,140.91
S$6327
  Bottom 0: 262.2,140.91 262.16,140.59
S$6328
  Bottom 0: 262.16,140.59 262.2,140.29
S$6329
  Bottom 0: 262.2,140.29 261.9,140
S$6330
  Bottom 0: 261.9,140 261.9,141.48
S$6331
  Bottom 0: 261.9,141.48 261.89,141.55
S$6332
  Bottom 0: 261.89,141.55 261.85,141.62
S$6333
  Bottom 0: 261.85,141.62 261.8,141.68
S$6334
  Bottom 0: 261.8,141.68 261.73,141.72
S$6335
  Bottom 0: 261.73,141.72 261.65,141.73
S$6336
  Bottom 0: 261.65,141.73 261.2,141.73
S$6337
  Bottom 0: 261.2,141.73 261.2,141.86
S$6338
  Bottom 0: 261.2,141.86 261.14,142.08
S$6339
  Bottom 0: 261.14,142.08 260.98,142.24
S$6340
  Bottom 0: 260.98,142.24 260.76,142.3
S$6341
  Bottom 0: 260.76,142.3 260.43,142.3
S$6342
  Bottom 0: 260.43,142.3 259.34,143.39
S$6343
  Bottom 0: 259.34,143.39 259.4,143.52
S$6344
  Bottom 0: 259.4,143.52 259.45,143.84
S$6345
  Bottom 0: 259.45,143.84 259.44,143.88
S$6346
  Bottom 0: 259.44,143.88 261.24,142.08
S$6347
  Bottom 0: 261.24,142.08 261.3,142.04
S$6348
  Bottom 0: 261.3,142.04 261.36,142
S$6349
  Bottom 0: 261.36,142 261.42,141.97
S$6350
  Bottom 0: 261.42,141.97 261.48,141.96
S$6351
  Bottom 0: 261.48,141.96 261.55,141.95
S$6352
  Bottom 0: 261.55,141.95 279.15,141.95
S$6353
  Bottom 0: 279.15,141.95 279.21,141.96
S$6354
  Bottom 0: 279.21,141.96 261.04,123.78
S$6355
  Bottom 0: 261.04,123.78 261,123.72
S$6356
  Bottom 0: 261,123.72 260.95,123.66
S$6357
  Bottom 0: 260.95,123.66 260.93,123.6
S$6358
  Bottom 0: 260.93,123.6 260.91,123.53
S$6359
  Bottom 0: 260.91,123.53 260.91,123.46
S$6360
  Bottom 0: 260.91,123.46 260.91,118.07
S$6361
  Bottom 0: 260.91,118.07 260.86,118.11
S$6362
  Bottom 0: 260.86,118.11 260.61,118.18
S$6363
  Bottom 0: 260.61,118.18 260.37,118.16
S$6364
  Bottom 0: 260.37,118.16 260.14,118.04
S$6365
  Bottom 0: 260.14,118.04 259.97,117.86
S$6366
  Bottom 0: 259.97,117.86 259.88,117.62
S$6367
  Bottom 0: 259.88,117.62 259.88,117.37
S$6368
  Bottom 0: 259.88,117.37 259.97,117.14
S$6369
  Bottom 0: 259.97,117.14 260.11,116.99
S$6370
  Bottom 0: 260.11,116.99 260.11,115.95
S$6371
  Bottom 0: 260.11,115.95 259.18,115.02
S$6372
  Bottom 0: 259.18,115.02 259.14,114.97
S$6373
  Bottom 0: 259.14,114.97 259.1,114.91
S$6374
  Bottom 0: 259.1,114.91 259.07,114.84
S$6375
  Bottom 0: 259.07,114.84 259.06,114.78
S$6376
  Bottom 0: 259.06,114.78 259.05,114.71
S$6377
  Bottom 0: 259.05,114.71 259.05,113.26
S$6378
  Bottom 0: 259.05,113.26 259.06,113.2
S$6379
  Bottom 0: 259.06,113.2 259.07,113.13
S$6380
  Bottom 0: 259.07,113.13 259.1,113.07
S$6381
  Bottom 0: 259.1,113.07 259.13,113.01
S$6382
  Bottom 0: 259.13,113.01 259.18,112.95
S$6383
  Bottom 0: 259.18,112.95 259.26,112.87
S$6384
  Bottom 0: 259.26,112.87 259.26,103.99
S$6385
  Bottom 0: 259.26,103.99 259.12,104.14
S$6386
  Bottom 0: 259.12,104.14 258.93,104.26
S$6387
  Bottom 0: 258.93,104.26 258.93,107.62
S$6388
  Bottom 0: 258.93,107.62 258.92,107.7
S$6389
  Bottom 0: 258.92,107.7 258.91,107.76
S$6390
  Bottom 0: 258.91,107.76 258.88,107.82
S$6391
  Bottom 0: 258.88,107.82 258.84,107.88
S$6392
  Bottom 0: 258.84,107.88 258.8,107.94
S$6393
  Bottom 0: 258.8,107.94 255.98,110.76
S$6394
  Bottom 0: 255.98,110.76 256.08,111.03
S$6395
  Bottom 0: 256.08,111.03 256.13,111.38
S$6396
  Bottom 0: 256.13,111.38 256.08,111.72
S$6397
  Bottom 0: 256.08,111.72 255.96,112.05
S$6398
  Bottom 0: 255.96,112.05 255.75,112.33
S$6399
  Bottom 0: 255.75,112.33 255.48,112.56
S$6400
  Bottom 0: 255.48,112.56 255.16,112.71
S$6401
  Bottom 0: 255.16,112.71 254.82,112.77
S$6402
  Bottom 0: 254.82,112.77 254.47,112.75
S$6403
  Bottom 0: 254.47,112.75 254.14,112.64
S$6404
  Bottom 0: 254.14,112.64 253.84,112.46
S$6405
  Bottom 0: 253.84,112.46 253.6,112.2
S$6406
  Bottom 0: 253.6,112.2 253.43,111.89
S$6407
  Bottom 0: 253.43,111.89 253.34,111.55
S$6408
  Bottom 0: 253.34,111.55 253.34,111.21
S$6409
  Bottom 0: 253.34,111.21 253.43,110.87
S$6410
  Bottom 0: 253.43,110.87 253.6,110.56
S$6411
  Bottom 0: 253.6,110.56 253.84,110.3
S$6412
  Bottom 0: 253.84,110.3 254.14,110.11
S$6413
  Bottom 0: 254.14,110.11 254.47,110.01
S$6414
  Bottom 0: 254.47,110.01 254.82,109.99
S$6415
  Bottom 0: 254.82,109.99 255.16,110.05
S$6416
  Bottom 0: 255.16,110.05 255.35,110.13
S$6417
  Bottom 0: 255.35,110.13 258.04,107.44
S$6418
  Bottom 0: 258.04,107.44 258.04,104.26
S$6419
  Bottom 0: 258.04,104.26 257.98,104.23
S$6420
  Bottom 0: 257.98,104.23 257.74,104.04
S$6421
  Bottom 0: 257.74,104.04 257.57,103.8
S$6422
  Bottom 0: 257.57,103.8 257.48,103.5
S$6423
  Bottom 0: 257.48,103.5 257.48,103.2
S$6424
  Bottom 0: 257.48,103.2 257.57,102.91
S$6425
  Bottom 0: 257.57,102.91 257.74,102.66
S$6426
  Bottom 0: 257.74,102.66 257.98,102.47
S$6427
  Bottom 0: 257.98,102.47 258.26,102.36
S$6428
  Bottom 0: 258.26,102.36 258.56,102.34
S$6429
  Bottom 0: 258.56,102.34 258.85,102.41
S$6430
  Bottom 0: 258.85,102.41 259.12,102.56
S$6431
  Bottom 0: 259.12,102.56 259.26,102.71
S$6432
  Bottom 0: 259.26,102.71 259.26,97.14
S$6433
  Bottom 0: 259.26,97.14 258.81,96.69
S$6434
  Bottom 0: 258.81,96.69 258.56,96.74
S$6435
  Bottom 0: 258.56,96.74 258.26,96.72
S$6436
  Bottom 0: 258.26,96.72 257.98,96.61
S$6437
  Bottom 0: 257.98,96.61 257.74,96.42
S$6438
  Bottom 0: 257.74,96.42 257.57,96.17
S$6439
  Bottom 0: 257.57,96.17 257.48,95.89
S$6440
  Bottom 0: 257.48,95.89 257.48,95.58
S$6441
  Bottom 0: 257.48,95.58 257.57,95.29
S$6442
  Bottom 0: 257.57,95.29 257.74,95.04
S$6443
  Bottom 0: 257.74,95.04 257.98,94.85
S$6444
  Bottom 0: 257.98,94.85 258.26,94.74
S$6445
  Bottom 0: 258.26,94.74 258.56,94.72
S$6446
  Bottom 0: 258.56,94.72 258.85,94.79
S$6447
  Bottom 0: 258.85,94.79 259.12,94.94
S$6448
  Bottom 0: 259.12,94.94 259.32,95.16
S$6449
  Bottom 0: 259.32,95.16 259.46,95.43
S$6450
  Bottom 0: 259.46,95.43 259.5,95.73
S$6451
  Bottom 0: 259.5,95.73 259.46,96.03
S$6452
  Bottom 0: 259.46,96.03 259.44,96.06
S$6453
  Bottom 0: 259.44,96.06 260.02,96.65
S$6454
  Bottom 0: 260.02,96.65 260.06,96.7
S$6455
  Bottom 0: 260.06,96.7 260.1,96.76
S$6456
  Bottom 0: 260.1,96.76 260.12,96.82
S$6457
  Bottom 0: 260.12,96.82 260.14,96.89
S$6458
  Bottom 0: 260.14,96.89 260.15,96.96
S$6459
  Bottom 0: 260.15,96.96 260.15,112.89
S$6460
  Bottom 0: 260.15,112.89 260.19,112.84
S$6461
  Bottom 0: 260.19,112.84 260.49,112.65
S$6462
  Bottom 0: 260.49,112.65 260.81,112.55
S$6463
  Bottom 0: 260.81,112.55 261.17,112.53
S$6464
  Bottom 0: 261.17,112.53 261.51,112.59
S$6465
  Bottom 0: 261.51,112.59 261.7,112.67
S$6466
  Bottom 0: 261.7,112.67 270.07,104.3
S$6467
  Bottom 0: 270.07,104.3 270.07,101.96
S$6468
  Bottom 0: 270.07,101.96 270.04,102.02
S$6469
  Bottom 0: 270.04,102.02 269.84,102.24
S$6470
  Bottom 0: 269.84,102.24 269.57,102.39
S$6471
  Bottom 0: 269.57,102.39 269.28,102.46
S$6472
  Bottom 0: 269.28,102.46 268.98,102.44
S$6473
  Bottom 0: 268.98,102.44 268.69,102.33
S$6474
  Bottom 0: 268.69,102.33 268.46,102.14
S$6475
  Bottom 0: 268.46,102.14 268.29,101.89
S$6476
  Bottom 0: 268.29,101.89 268.2,101.6
S$6477
  Bottom 0: 268.2,101.6 268.2,101.3
S$6478
  Bottom 0: 268.2,101.3 268.25,101.12
S$6479
  Bottom 0: 268.25,101.12 260.81,93.68
S$6480
  Bottom 0: 260.81,93.68 256.54,93.68
S$6481
  Bottom 0: 256.54,93.68 256.66,93.72
S$6482
  Bottom 0: 256.66,93.72 256.92,93.91
S$6483
  Bottom 0: 256.92,93.91 257.13,94.16
S$6484
  Bottom 0: 257.13,94.16 257.26,94.46
S$6485
  Bottom 0: 257.26,94.46 257.3,94.78
S$6486
  Bottom 0: 257.3,94.78 257.26,95.1
S$6487
  Bottom 0: 257.26,95.1 257.13,95.4
S$6488
  Bottom 0: 257.13,95.4 256.92,95.66
S$6489
  Bottom 0: 256.92,95.66 256.66,95.84
S$6490
  Bottom 0: 256.66,95.84 256.35,95.95
S$6491
  Bottom 0: 256.35,95.95 256.03,95.97
S$6492
  Bottom 0: 256.03,95.97 255.71,95.91
S$6493
  Bottom 0: 255.71,95.91 255.42,95.76
S$6494
  Bottom 0: 255.42,95.76 255.18,95.53
S$6495
  Bottom 0: 255.18,95.53 255.01,95.26
S$6496
  Bottom 0: 255.01,95.26 254.93,94.94
S$6497
  Bottom 0: 254.93,94.94 254.93,94.62
S$6498
  Bottom 0: 254.93,94.62 255.01,94.31
S$6499
  Bottom 0: 255.01,94.31 255.18,94.03
S$6500
  Bottom 0: 255.18,94.03 255.42,93.81
S$6501
  Bottom 0: 255.42,93.81 255.67,93.68
S$6502
  Bottom 0: 255.67,93.68 252.28,93.68
S$6503
  Bottom 0: 265.93,131.58 266.27,131.64
S$6504
  Bottom 0: 266.27,131.64 266.59,131.79
S$6505
  Bottom 0: 266.59,131.79 266.86,132.01
S$6506
  Bottom 0: 266.86,132.01 267.07,132.3
S$6507
  Bottom 0: 267.07,132.3 267.19,132.62
S$6508
  Bottom 0: 267.19,132.62 267.24,132.97
S$6509
  Bottom 0: 267.24,132.97 267.19,133.31
S$6510
  Bottom 0: 267.19,133.31 267.09,133.58
S$6511
  Bottom 0: 267.09,133.58 272.97,139.46
S$6512
  Bottom 0: 272.97,139.46 273.07,139.46
S$6513
  Bottom 0: 273.07,139.46 273.31,139.52
S$6514
  Bottom 0: 273.31,139.52 273.51,139.68
S$6515
  Bottom 0: 273.51,139.68 273.65,139.89
S$6516
  Bottom 0: 273.65,139.89 273.69,140.14
S$6517
  Bottom 0: 273.69,140.14 273.65,140.39
S$6518
  Bottom 0: 273.65,140.39 273.51,140.6
S$6519
  Bottom 0: 273.51,140.6 273.31,140.75
S$6520
  Bottom 0: 273.31,140.75 273.07,140.82
S$6521
  Bottom 0: 273.07,140.82 272.82,140.79
S$6522
  Bottom 0: 272.82,140.79 272.6,140.69
S$6523
  Bottom 0: 272.6,140.69 272.43,140.5
S$6524
  Bottom 0: 272.43,140.5 272.33,140.26
S$6525
  Bottom 0: 272.33,140.26 272.33,140.09
S$6526
  Bottom 0: 272.33,140.09 266.46,134.21
S$6527
  Bottom 0: 266.46,134.21 266.27,134.3
S$6528
  Bottom 0: 266.27,134.3 265.93,134.36
S$6529
  Bottom 0: 265.93,134.36 265.58,134.34
S$6530
  Bottom 0: 265.58,134.34 265.25,134.23
S$6531
  Bottom 0: 265.25,134.23 264.95,134.05
S$6532
  Bottom 0: 264.95,134.05 264.71,133.79
S$6533
  Bottom 0: 264.71,133.79 264.54,133.48
S$6534
  Bottom 0: 264.54,133.48 264.45,133.14
S$6535
  Bottom 0: 264.45,133.14 264.45,132.79
S$6536
  Bottom 0: 264.45,132.79 264.54,132.46
S$6537
  Bottom 0: 264.54,132.46 264.71,132.15
S$6538
  Bottom 0: 264.71,132.15 264.95,131.89
S$6539
  Bottom 0: 264.95,131.89 265.25,131.7
S$6540
  Bottom 0: 265.25,131.7 265.58,131.6
S$6541
  Bottom 0: 265.58,131.6 265.93,131.58
S$6542
  Bottom 0: 105.45,93.85
S$6543
  Bottom 0: 105.45,93.85 111.38,99.78
S$6544
  Bottom 0: 111.38,99.78 111.42,99.84
S$6545
  Bottom 0: 111.42,99.84 111.46,99.9
S$6546
  Bottom 0: 111.46,99.9 111.48,99.96
S$6547
  Bottom 0: 111.48,99.96 111.5,100.03
S$6548
  Bottom 0: 111.5,100.03 111.51,100.1
S$6549
  Bottom 0: 111.51,100.1 111.51,112.59
S$6550
  Bottom 0: 111.51,112.59 111.81,112.74
S$6551
  Bottom 0: 111.81,112.74 112.08,112.96
S$6552
  Bottom 0: 112.08,112.96 112.29,113.25
S$6553
  Bottom 0: 112.29,113.25 112.42,113.57
S$6554
  Bottom 0: 112.42,113.57 112.46,113.92
S$6555
  Bottom 0: 112.46,113.92 112.42,114.26
S$6556
  Bottom 0: 112.42,114.26 112.29,114.59
S$6557
  Bottom 0: 112.29,114.59 112.08,114.87
S$6558
  Bottom 0: 112.08,114.87 111.81,115.1
S$6559
  Bottom 0: 111.81,115.1 111.5,115.25
S$6560
  Bottom 0: 111.5,115.25 111.15,115.31
S$6561
  Bottom 0: 111.15,115.31 110.8,115.29
S$6562
  Bottom 0: 110.8,115.29 110.5,115.19
S$6563
  Bottom 0: 110.5,115.19 111.48,116.17
S$6564
  Bottom 0: 111.48,116.17 111.54,116.23
S$6565
  Bottom 0: 111.54,116.23 111.58,116.31
S$6566
  Bottom 0: 111.58,116.31 111.62,116.39
S$6567
  Bottom 0: 111.62,116.39 111.64,116.48
S$6568
  Bottom 0: 111.64,116.48 111.64,116.57
S$6569
  Bottom 0: 111.64,116.57 111.64,123.75
S$6570
  Bottom 0: 111.64,123.75 111.89,123.92
S$6571
  Bottom 0: 111.89,123.92 112.09,124.18
S$6572
  Bottom 0: 112.09,124.18 112.22,124.47
S$6573
  Bottom 0: 112.22,124.47 112.27,124.8
S$6574
  Bottom 0: 112.27,124.8 112.22,125.11
S$6575
  Bottom 0: 112.22,125.11 112.09,125.42
S$6576
  Bottom 0: 112.09,125.42 111.89,125.67
S$6577
  Bottom 0: 111.89,125.67 111.71,125.79
S$6578
  Bottom 0: 111.71,125.79 112.31,125.79
S$6579
  Bottom 0: 112.31,125.79 112.38,125.8
S$6580
  Bottom 0: 112.38,125.8 112.45,125.81
S$6581
  Bottom 0: 112.45,125.81 112.51,125.84
S$6582
  Bottom 0: 112.51,125.84 112.56,125.88
S$6583
  Bottom 0: 112.56,125.88 112.62,125.92
S$6584
  Bottom 0: 112.62,125.92 116.96,130.25
S$6585
  Bottom 0: 116.96,130.25 117,130.31
S$6586
  Bottom 0: 117,130.31 117.04,130.37
S$6587
  Bottom 0: 117.04,130.37 117.07,130.43
S$6588
  Bottom 0: 117.07,130.43 117.08,130.5
S$6589
  Bottom 0: 117.08,130.5 117.09,130.57
S$6590
  Bottom 0: 117.09,130.57 117.09,131.68
S$6591
  Bottom 0: 117.09,131.68 122.27,136.85
S$6592
  Bottom 0: 122.27,136.85 122.31,136.91
S$6593
  Bottom 0: 122.31,136.91 122.35,136.96
S$6594
  Bottom 0: 122.35,136.96 122.38,137.03
S$6595
  Bottom 0: 122.38,137.03 122.39,137.09
S$6596
  Bottom 0: 122.39,137.09 122.4,137.16
S$6597
  Bottom 0: 122.4,137.16 122.4,145.88
S$6598
  Bottom 0: 122.4,145.88 122.39,145.95
S$6599
  Bottom 0: 122.39,145.95 122.38,146.02
S$6600
  Bottom 0: 122.38,146.02 122.35,146.08
S$6601
  Bottom 0: 122.35,146.08 122.31,146.14
S$6602
  Bottom 0: 122.31,146.14 122.27,146.19
S$6603
  Bottom 0: 122.27,146.19 117.07,151.4
S$6604
  Bottom 0: 117.07,151.4 117.17,151.67
S$6605
  Bottom 0: 117.17,151.67 117.22,152.02
S$6606
  Bottom 0: 117.22,152.02 117.17,152.36
S$6607
  Bottom 0: 117.17,152.36 117.05,152.69
S$6608
  Bottom 0: 117.05,152.69 116.84,152.97
S$6609
  Bottom 0: 116.84,152.97 116.57,153.2
S$6610
  Bottom 0: 116.57,153.2 116.27,153.34
S$6611
  Bottom 0: 116.27,153.34 116.27,154.28
S$6612
  Bottom 0: 116.27,154.28 116.26,154.35
S$6613
  Bottom 0: 116.26,154.35 116.25,154.41
S$6614
  Bottom 0: 116.25,154.41 116.22,154.48
S$6615
  Bottom 0: 116.22,154.48 116.18,154.53
S$6616
  Bottom 0: 116.18,154.53 116.13,154.59
S$6617
  Bottom 0: 116.13,154.59 112.69,158.03
S$6618
  Bottom 0: 112.69,158.03 112.64,158.07
S$6619
  Bottom 0: 112.64,158.07 112.58,158.11
S$6620
  Bottom 0: 112.58,158.11 112.52,158.13
S$6621
  Bottom 0: 112.52,158.13 112.45,158.15
S$6622
  Bottom 0: 112.45,158.15 112.38,158.16
S$6623
  Bottom 0: 112.38,158.16 110.48,158.16
S$6624
  Bottom 0: 110.48,158.16 110.14,158.5
S$6625
  Bottom 0: 110.14,158.5 111.63,158.5
S$6626
  Bottom 0: 111.63,158.5 111.71,158.51
S$6627
  Bottom 0: 111.71,158.51 111.78,158.55
S$6628
  Bottom 0: 111.78,158.55 111.83,158.6
S$6629
  Bottom 0: 111.83,158.6 111.88,158.67
S$6630
  Bottom 0: 111.88,158.67 111.89,158.75
S$6631
  Bottom 0: 111.89,158.75 111.89,160.53
S$6632
  Bottom 0: 111.89,160.53 111.88,160.6
S$6633
  Bottom 0: 111.88,160.6 111.83,160.68
S$6634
